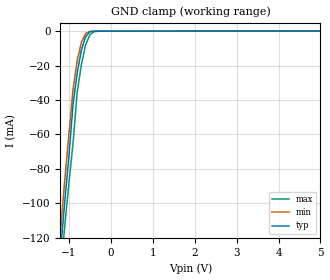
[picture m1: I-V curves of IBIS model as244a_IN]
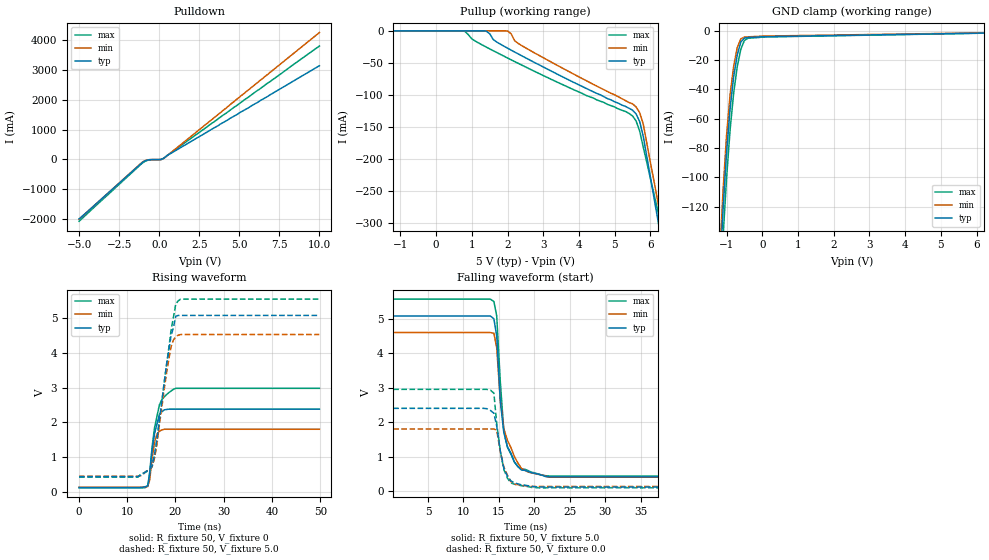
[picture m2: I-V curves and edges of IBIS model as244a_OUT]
| TEXAS INSTRUMENTS INCORPORATED
| Standard Linear and Logic Group
| IBIS Model of SN74AS244A
| OCTAL BUFFERS AND LINE DRIVERS WITH 3-STATE OUTPUTS
| SOP 20-pin (NS), SSOP 20-pin (DB), SOIC 20-pin (DW), PDIP 20-pin (N) Packages
[IBIS Ver]   3.2
[Comment Char]  |_char
[File Name]   sn74as244a.ibs
[File Rev]   2.1 I_die
[Date]   Sept. 30, 2004
[Source]   File originated at Texas Instruments, Inc.
[Notes]   The following is a sample IBIS file for the AS244A.
   - FILE REV HISTORY
   - 2.1 Re-Release IBIS file on 10/08/04
   - Power clamp data deleted as there is no power-clamp diode
|   - All test data contained in this file are derived from
|   actual measurements.
|   - File created by Nobuhisa Ohtsubo, SLL Product Engineering.
[Disclaimer] Property of Texas Instruments Incorporated.  Unauthorized
   reproduction and/or distribution is strictly prohibited.
   This product is protected under copyright law.
   Created 2000, (C) Copyright 2000, Texas Instruments Inc.,
   All Rights Reserved.
   UNLESS THERE IS A SIGNED, WRITTEN AGREEMENT TO THE
   CONTRARY, TEXAS INSTRUMENTS () IS PROVIDING THE IBIS
   MODELS  AND WITHOUT ANY WARRANTY, EXPRESSED OR
   IMPLIED.  TI assumes no liability for:
   1) the accuracy of the IBIS models provided to your
   company;
   2) the proper functioning of these IBIS Models in your
   design or for any resulting applications; or
   3) infringement of patents, copyrights or intellectual
   property rights resulting from your use of these IBIS
   models.
   TI provides IBIS Models as a service to our customers.
   You and your company shall not distribute, sell or give
   these models to anyone else without prior written
   permission from TI.
   TI reserves the right to make changes to our products or
   to discontinue any semiconductor product or service
   without notice, and advises our customers to obtain the
   latest version of relevant information to verify, before
   placing orders, that the information being relied on is
   current.
   Please be aware that your receipt and use of the IBIS
   information provided shall serve as acceptance of these
   terms and conditions.  If you do not accept these terms,
   you should return or destroy the IBIS models and any
   other accompanying information immediately.
|   Component AS244A_NS
[Component]   as244a_NS
[Manufacturer]  Texas Instruments, Inc.
[Package]
|   typ   min   max
R_pkg   0.044   0.029   0.058
L_pkg   3.666nH   2.317nH   5.115nH
C_pkg   0.548pF   0.316pF   0.725pF
[Pin]   signal_name   model_name   R_pin   L_pin   C_pin
1   1OE_NOT   as244a_IN   0.058   5.115nH   0.725pF
2   1A1   as244a_IN   0.053   4.591nH   0.724pF
3   2Y4   as244a_OUT   0.049   3.754nH   0.572pF
4   1A2   as244a_IN   0.029   2.549nH   0.388pF
5   2Y3   as244a_OUT   0.031   2.317nH   0.316pF
6   1A3   as244a_IN   0.031   2.317nH   0.316pF
7   2Y2   as244a_OUT   0.029   2.556nH   0.399pF
8   1A4   as244a_IN   0.049   3.754nH   0.579pF
9   2Y1   as244a_OUT   0.053   4.591nH   0.724pF
10   GND   GND   0.058   5.115nH   0.725pF
11   2A1   as244a_IN   0.058   5.115nH   0.725pF
12   1Y4   as244a_OUT   0.053   4.591nH   0.724pF
13   2A2   as244a_IN   0.049   3.754nH   0.579pF
14   1Y3   as244a_OUT   0.029   2.557nH   0.399pF
15   2A3   as244a_IN   0.031   2.317nH   0.316pF
16   1Y2   as244a_OUT   0.031   2.317nH   0.316pF
17   2A4   as244a_IN   0.029   2.557nH   0.399pF
18   1Y1   as244a_OUT   0.049   3.754nH   0.579pF
19   2OE_NOT   as244a_IN   0.053   4.591nH   0.724pF
20   VCC   POWER   0.058   5.115nH   0.725pF
|   Component AS244A_DB
[Component]   as244a_DB
[Manufacturer]  Texas Instruments, Inc.
[Package]
|   typ   min   max
R_pkg   0.040   0.035   0.051
L_pkg   3.495nH   3.035nH   4.314nH
C_pkg   0.420pF   0.346pF   0.502pF
[Pin]   signal_name   model_name   R_pin   L_pin   C_pin
1   1OE_NOT   as244a_IN   0.049   4.310nH   0.502pF
2   1A1   as244a_IN   0.048   3.903nH   0.487pF
3   2Y4   as244a_OUT   0.035   3.189nH   0.396pF
4   1A2   as244a_IN   0.035   3.036nH   0.347pF
5   2Y3   as244a_OUT   0.035   3.035nH   0.367pF
6   1A3   as244a_IN   0.035   3.035nH   0.367pF
7   2Y2   as244a_OUT   0.035   3.036nH   0.347pF
8   1A4   as244a_IN   0.035   3.189nH   0.397pF
9   2Y1   as244a_OUT   0.047   3.899nH   0.488pF
10   GND   GND   0.051   4.314nH   0.500pF
11   2A1   as244a_IN   0.051   4.314nH   0.500pF
12   1Y4   as244a_OUT   0.047   3.899nH   0.488pF
13   2A2   as244a_IN   0.035   3.189nH   0.397pF
14   1Y3   as244a_OUT   0.035   3.036nH   0.346pF
15   2A3   as244a_IN   0.035   3.035nH   0.367pF
16   1Y2   as244a_OUT   0.035   3.035nH   0.367pF
17   2A4   as244a_IN   0.035   3.036nH   0.346pF
18   1Y1   as244a_OUT   0.035   3.189nH   0.397pF
19   2OE_NOT   as244a_IN   0.047   3.899nH   0.488pF
20   VCC   POWER   0.051   4.314nH   0.502pF
|   Component as244a_DW
[Component]   as244a_DW
[Manufacturer]   Texas Instruments, Inc.
[Package]
|   typ   min   max
R_pkg   3.800e-02   3.300e-02   4.500e-02
L_pkg   5.012e-09   4.110e-09   6.349e-09
C_pkg   7.170e-13   5.300e-13   8.680e-13
[Pin]   signal_name   model_name   R_pin   L_pin   C_pin
1   1OE_NOT   as244a_IN   4.200e-02   6.336e-09   8.650e-13
2   1A1   as244a_IN   4.300e-02   5.542e-09   8.670e-13
3   2Y4   as244a_OUT   3.400e-02   4.714e-09   7.320e-13
4   1A2   as244a_IN   3.400e-02   4.377e-09   5.910e-13
5   2Y3   as244a_OUT   3.600e-02   4.130e-09   5.330e-13
6   1A3   as244a_IN   3.500e-02   4.111e-09   5.300e-13
7   2Y2   as244a_OUT   3.400e-02   4.284e-09   5.830e-13
8   1A4   as244a_IN   3.400e-02   4.634e-09   7.260e-13
9   2Y1   as244a_OUT   4.000e-02   5.518e-09   8.650e-13
10   GND   GND   4.300e-02   6.349e-09   8.660e-13
11   2A1   as244a_IN   4.100e-02   6.281e-09   8.610e-13
12   1Y4   as244a_OUT   4.500e-02   5.561e-09   8.680e-13
13   2A2   as244a_IN   3.300e-02   4.778e-09   7.420e-13
14   1Y3   as244a_OUT   3.500e-02   4.414e-09   5.960e-13
15   2A3   as244a_IN   3.500e-02   4.110e-09   5.330e-13
16   1Y2   as244a_OUT   3.600e-02   4.130e-09   5.330e-13
17   2A4   as244a_IN   3.400e-02   4.377e-09   5.910e-13
18   1Y1   as244a_OUT   3.400e-02   4.714e-09   7.310e-13
19   2OE_NOT   as244a_IN   4.300e-02   5.569e-09   8.680e-13
20   VCC   POWER   4.200e-02   6.308e-09   8.640e-13
|   Component as244a_N
[Component]   as244a_N
[Manufacturer]   Texas Instruments, Inc.
[Package]
|   typ   min   max
R_pkg   4.300e-02   3.800e-02   5.000e-02
L_pkg   7.384e-09   4.680e-09   1.032e-08
C_pkg   5.100e-13   2.310e-13   8.210e-13
[Pin]   signal_name   model_name   R_pin   L_pin   C_pin
1   1OE_NOT   as244a_IN   4.200e-02   9.427e-09   8.100e-13
2   1A1   as244a_IN   4.600e-02   8.544e-09   4.560e-13
3   2Y4   as244a_OUT   4.800e-02   7.163e-09   4.350e-13
4   1A2   as244a_IN   4.000e-02   4.825e-09   2.610e-13
5   2Y3   as244a_OUT   4.000e-02   5.284e-09   6.480e-13
6   1A3   as244a_IN   4.000e-02   4.686e-09   2.320e-13
7   2Y2   as244a_OUT   4.000e-02   6.359e-09   4.890e-13
8   1A4   as244a_IN   3.800e-02   7.982e-09   4.750e-13
9   2Y1   as244a_OUT   4.300e-02   9.403e-09   4.750e-13
10   GND   GND   5.000e-02   1.032e-08   8.050e-13
11   2A1   as244a_IN   5.000e-02   1.028e-08   8.100e-13
12   1Y4   as244a_OUT   4.300e-02   9.383e-09   4.770e-13
13   2A2   as244a_IN   3.800e-02   7.978e-09   4.760e-13
14   1Y3   as244a_OUT   4.000e-02   6.302e-09   4.920e-13
15   2A3   as244a_IN   4.000e-02   4.680e-09   2.310e-13
16   1Y2   as244a_OUT   4.000e-02   5.284e-09   6.480e-13
17   2A4   as244a_IN   4.000e-02   4.822e-09   2.610e-13
18   1Y1   as244a_OUT   4.700e-02   7.118e-09   4.390e-13
19   2OE_NOT   as244a_IN   4.600e-02   8.492e-09   4.610e-13
20   VCC   POWER   4.300e-02   9.348e-09   8.210e-13
| Models and submodels in the file (2): as244a_IN (Input), as244a_OUT (3-state)
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|   Model AS244A_IN
[Model]   as244a_IN
Model_type  Input
Polarity   Inverting
Vinl = 0.8
Vinh = 2.0
| variable   typ   min   max
C_comp   1.33pf   1.00pf   1.66pf
[Temperature Range]   25   0   70
[Voltage Range]   5.0   4.5   5.5
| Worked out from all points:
|   GND clamp passes 1 mA (typ) near -0.52 V on its own axis
[GND Clamp]
|   Voltage   I(typ)   I(min)   I(max)
-5V       -1.38A     -1.52A     -1.25A
-1.2V     -129mA     -117mA     -142mA
-1.1V     -99.9mA    -87.3mA    -114mA
-1V       -73.3mA    -60.3mA    -88.9mA
-900mV    -42.7mA    -33.9mA    -65.3mA
-800mV    -24.3mA    -17.1mA    -35.4mA
-700mV    -10.9mA    -6.51mA    -19.4mA
-600mV    -3.35mA    -1.4mA     -8.1mA
-500mV    -463uA     -155uA     -2.22mA
-400mV    -107uA     -95.3uA    -312uA
-300mV    -89uA      -90uA      -95.2uA
5V        281pA      4.14pA     442pA
|   Model AS244A_OUT
[Model]   as244a_OUT
Model_type  3-state
Polarity   Non-Inverting
Enable   Active-Low
Vmeas = 1.3v
Cref = 0pf
| variable   typ   min   max
C_comp   5.8pf   4.35pf   7.25pf
[Temperature Range]   25   0   70
[Voltage Range]   5.0   4.5   5.5
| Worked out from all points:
|   slope of the pulldown table from 0 to 0.75 V, typ, clamps not added: 3.5 ohm
|   rising waveform, R_fixture 50, V_fixture 0: 20-80 % time 1.41ns typ, 996ps min, 1.77ns max; typ from 0.121 V to 2.38 V
|   falling waveform, R_fixture 50, V_fixture 5.0: 20-80 % time 1.34ns typ, 1.91ns min, 1.16ns max; typ from 5.08 V to 0.411 V
|   rising waveform, R_fixture 50, V_fixture 5.0: 20-80 % time 2.71ns typ, 2.46ns min, 2.81ns max; typ from 0.433 V to 5.08 V
|   falling waveform, R_fixture 50, V_fixture 0.0: 20-80 % time 1.27ns typ, 1.26ns min, 1.16ns max; typ from 2.4 V to 0.115 V
[Pulldown]
|   Voltage   I(typ)   I(min)   I(max)
-5V       -1.99A     -2A        -2.07A
-1V       -83.4mA    -71.5mA    -101mA
-700mV    -16.4mA    -11.4mA    -24.3mA
100mV     -2.14mA    -2.67mA    -572uA
300mV     47.8mA     42.5mA     52.5mA
600mV     169mA      172mA      172mA
10V       3.14A      4.25A      3.8A
[Pullup]
|   Voltage   II(typ)   I(min)   I(max)
-5V       136nA      6.94nA     1.38uA
800mV     136nA      6.86nA     -582uA
1.4V      -285uA     6.69nA     -25.3mA
2V        -27.1mA    -212uA     -42.5mA
2.5V      -42mA      -26.5mA    -56.3mA
5.3V      -118mA     -109mA     -126mA
5.6V      -130mA     -119mA     -141mA
5.8V      -165mA     -146mA     -182mA
6.2V      -293mA     -265mA     -280mA
6.3V      -325mA     -295mA     -304mA
6.4V      -357mA     -325mA     -329mA
10V       -1.51A     -1.4A      -1.21A
[GND Clamp]
|   Voltage   I(typ)   I(min)   I(max)
-5V       -1.99A     -2A        -2.07A
-1.2V     -171mA     -159mA     -191mA
-1.1V     -123mA     -110mA     -142mA
-1V       -83.4mA    -71.5mA    -101mA
-900mV    -53mA      -43.4mA    -67.4mA
-800mV    -31.1mA    -24.1mA    -42.4mA
-700mV    -16.4mA    -11.4mA    -24.3mA
-600mV    -7.67mA    -5.42mA    -12.6mA
-500mV    -4.88mA    -4.25mA    -6.55mA
-400mV    -4.55mA    -4.1mA     -5.06mA
0V        -4.01mA    -3.6mA     -4.21mA
10V       10.1uA     16uA       12.1uA
[Ramp]
| variable   typ   min   max
dV/dt_r   1.692/2.512n   1.440/2.599n   1.890/2.454n
dV/dt_f   2.736/1.964n   2.442/2.271n   3.018/1.645n
R_load = 50
[Rising Waveform]
R_fixture = 50
V_fixture = 0
|   Time   V(typ)   V(min)   V(max)
97.7ps    121mV      130mV      111mV
14.3ns    166mV      149mV      174mV
14.7ns    499mV      340mV      556mV
15.2ns    1.2V       959mV      1.29V
15.7ns    1.67V      1.42V      1.84V
16.2ns    1.95V      1.66V      2.17V
16.7ns    2.22V      1.74V      2.5V
17.7ns    2.36V      1.8V       2.73V
20.1ns    2.38V      1.8V       2.98V
49.8ns    2.38V      1.8V       2.98V
[Falling Waveform]
R_fixture = 50
V_fixture = 5.0
V_fixture_min = 4.5
V_fixture_max = 5.5
|   Time   V(typ)   V(min)   V(max)
97.7ps    5.08V      4.6V       5.57V
14.3ns    5V         4.58V      5.5V
14.7ns    4.5V       4.16V      5.08V
15.2ns    2.63V      2.65V      3.19V
15.7ns    1.7V       1.81V      1.75V
16.2ns    1.29V      1.48V      1.28V
17.2ns    843mV      996mV      836mV
18.2ns    607mV      654mV      639mV
22.1ns    411mV      400mV      435mV
49.8ns    411mV      400mV      435mV
[Rising Waveform]
R_fixture = 50
V_fixture = 5.0
V_fixture_min = 4.5
V_fixture_max = 5.5
|   Time   V(typ)   V(min)   V(max)
97.7ps    433mV      445mV      423mV
12.3ns    438mV      445mV      423mV
15.2ns    746mV      729mV      719mV
15.7ns    1.07V      971mV      1.01V
16.2ns    1.51V      1.36V      1.46V
17.7ns    3.14V      2.95V      3.14V
19.1ns    4.48V      4.17V      4.64V
20.1ns    5.06V      4.47V      5.41V
20.6ns    5.08V      4.51V      5.5V
49.8ns    5.08V      4.53V      5.55V
[Falling Waveform]
R_fixture = 50
V_fixture = 0.0
|   Time   V(typ)   V(min)   V(max)
97.7ps    2.4V       1.8V       2.95V
13.8ns    2.34V      1.8V       2.93V
14.3ns    2.26V      1.8V       2.84V
14.7ns    1.88V      1.76V      1.95V
15.2ns    1.17V      1.15V      1.17V
15.7ns    667mV      699mV      625mV
16.7ns    291mV      268mV      231mV
17.2ns    238mV      199mV      197mV
21.1ns    116mV      130mV      91mV
49.8ns    115mV      130mV      92mV
